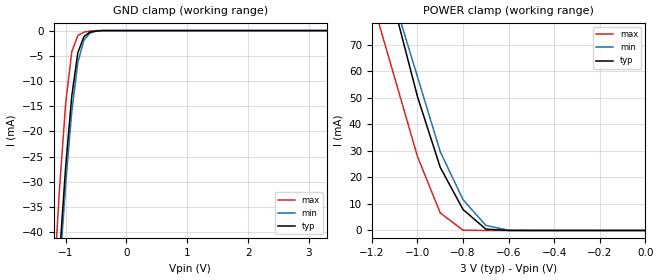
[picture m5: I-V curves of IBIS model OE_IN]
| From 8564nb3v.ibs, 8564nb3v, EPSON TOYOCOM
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[Model]   OE_IN
Model_type   Input
Polarity   Non-Inverting
Vinl =   0.9V
Vinh =   2.1V
C_comp   5pF   5pF   5pF
[Temperature Range]   25.00   85.00   -40.00
[Voltage Range]   3.0V   2.7V   3.3V
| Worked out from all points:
|   GND clamp passes 1 mA (typ) near -0.68 V on its own axis
|   POWER clamp passes 1 mA (typ) near -0.71 V on its own axis
[GND_clamp]
| voltage   I(typ)   I(min)   I(max)
-3.3V     -464.8mA   -454.9mA   -472mA
-1.2V     -63.5mA    -66.2mA    -51.2mA
-1.1V     -44.4mA    -47.6mA    -31.1mA
-1V       -27mA      -30.5mA    -14.4mA
-900mV    -13mA      -16.1mA    -4.2mA
-800mV    -4.4mA     -6.3mA     -1mA
-700mV    -1.2mA     -1.9mA     -300uA
-600mV    -300uA     -500uA     -100uA
-500mV    -100uA     -100uA     0A
-400mV    0A         0A         0A
3.3V      0A         0A         0A
[POWER_clamp]
| voltage   I(typ)   I(min)   I(max)
-3.3V     813.4mA    707.7mA    709.9mA
-1.2V     116.9mA    114.5mA    87.2mA
-1.1V     83.7mA     86.2mA     57.6mA
-1V       50.5mA     58mA       27.9mA
-900mV    23.8mA     29.7mA     6.6mA
-800mV    7.9mA      11.6mA     100uA
-700mV    500uA      1.9mA      0A
-600mV    0A         100uA      0A
0V        0A         0A         0A
